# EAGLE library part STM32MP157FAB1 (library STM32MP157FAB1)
32-bit Microcontrollers - MCU 16/32-BITS MICROS Source: Datasheet
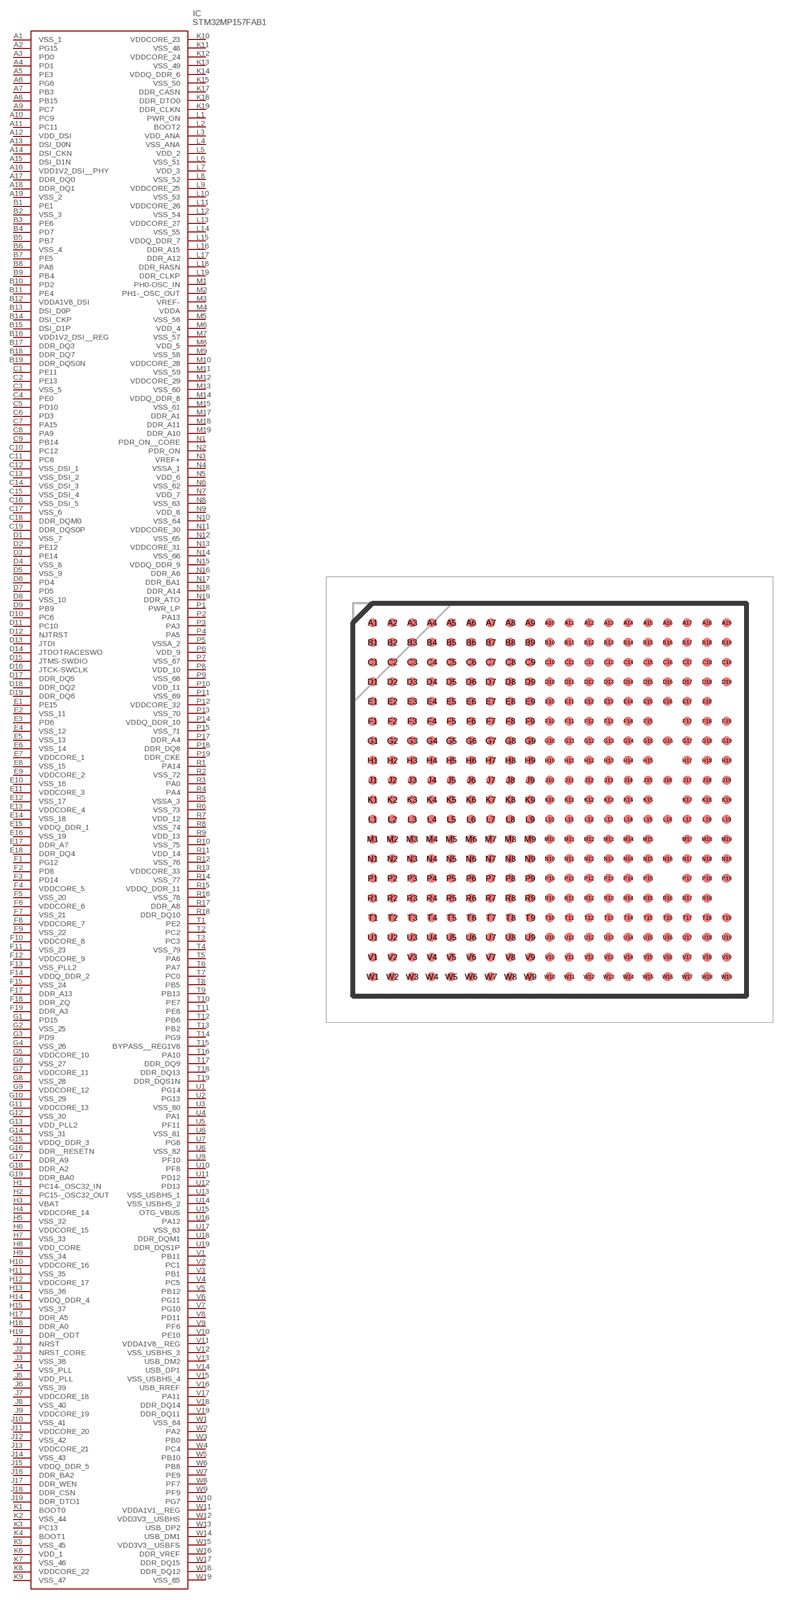
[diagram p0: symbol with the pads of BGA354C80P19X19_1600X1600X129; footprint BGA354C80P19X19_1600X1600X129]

Designator prefix IC

## STM32MP157FAB1 (Description: 32-bit Microcontrollers - MCU 16/32-BITS MICROS; Height: 1.29mm; Manufacturer_Name: STMicroelectronics; Manufacturer_Part_Number: STM32MP157FAB1; Mouser_Part_Number: 511-STM32MP157FAB1; Mouser_Price-Stock: https://www.mouser.co.uk/ProductDetail/STMicroelectronics/STM32MP157FAB1?qs=xZ%2FP%252Ba9zWqaMNhk4KMq8KA%3D%3D)  [BGA354C80P19X19_1600X1600X129]
A1  VSS_1
A2  PG15
A3  PD0
A4  PD1
A5  PE3
A6  PG6
A7  PB3
A8  PB15
A9  PC7
A10  PC9
A11  PC11
A12  VDD_DSI
A13  DSI_D0N
A14  DSI_CKN
A15  DSI_D1N
A16  VDD1V2_DSI__PHY
A17  DDR_DQ0
A18  DDR_DQ1
A19  VSS_2
B1  PE1
B2  VSS_3
B3  PE6
B4  PD7
B5  PB7
B6  VSS_4
B7  PE5
B8  PA8
B9  PB4
B10  PD2
B11  PE4
B12  VDDA1V8_DSI
B13  DSI_D0P
B14  DSI_CKP
B15  DSI_D1P
B16  VDD1V2_DSI__REG
B17  DDR_DQ3
B18  DDR_DQ7
B19  DDR_DQS0N
C1  PE11
C2  PE13
C3  VSS_5
C4  PE0
C5  PD10
C6  PD3
C7  PA15
C8  PA9
C9  PB14
C10  PC12
C11  PC8
C12  VSS_DSI_1
C13  VSS_DSI_2
C14  VSS_DSI_3
C15  VSS_DSI_4
C16  VSS_DSI_5
C17  VSS_6
C18  DDR_DQM0
C19  DDR_DQS0P
D1  VSS_7
D2  PE12
D3  PE14
D4  VSS_8
D5  VSS_9
D6  PD4
D7  PD5
D8  VSS_10
D9  PB9
D10  PC6
D11  PC10
D12  NJTRST
D13  JTDI
D14  JTDOTRACESWO
D15  JTMS-SWDIO
D16  JTCK-SWCLK
D17  DDR_DQ5
D18  DDR_DQ2
D19  DDR_DQ6
E1  PE15
E2  VSS_11
E3  PD6
E4  VSS_12
E5  VSS_13
E6  VSS_14
E7  VDDCORE_1
E8  VSS_15
E9  VDDCORE_2
E10  VSS_16
E11  VDDCORE_3
E12  VSS_17
E13  VDDCORE_4
E14  VSS_18
E15  VDDQ_DDR_1
E16  VSS_19
E17  DDR_A7
E18  DDR_DQ4
F1  PG12
F2  PD8
F3  PD14
F4  VDDCORE_5
F5  VSS_20
F6  VDDCORE_6
F7  VSS_21
F8  VDDCORE_7
F9  VSS_22
F10  VDDCORE_8
F11  VSS_23
F12  VDDCORE_9
F13  VSS_PLL2
F14  VDDQ_DDR_2
F15  VSS_24
F17  DDR_A13
F18  DDR_ZQ
F19  DDR_A3
G1  PD15
G2  VSS_25
G3  PD9
G4  VSS_26
G5  VDDCORE_10
G6  VSS_27
G7  VDDCORE_11
G8  VSS_28
G9  VDDCORE_12
G10  VSS_29
G11  VDDCORE_13
G12  VSS_30
G13  VDD_PLL2
G14  VSS_31
G15  VDDQ_DDR_3
G16  DDR__RESETN
G17  DDR_A9
G18  DDR_A2
G19  DDR_BA0
H1  PC14-_OSC32_IN
H2  PC15-_OSC32_OUT
H3  VBAT
H4  VDDCORE_14
H5  VSS_32
H6  VDDCORE_15
H7  VSS_33
H8  VDD_CORE
H9  VSS_34
H10  VDDCORE_16
H11  VSS_35
H12  VDDCORE_17
H13  VSS_36
H14  VDDQ_DDR_4
H15  VSS_37
H17  DDR_A5
H18  DDR_A0
H19  DDR__ODT
J1  NRST
J2  NRST_CORE
J3  VSS_38
J4  VSS_PLL
J5  VDD_PLL
J6  VSS_39
J7  VDDCORE_18
J8  VSS_40
J9  VDDCORE_19
J10  VSS_41
J11  VDDCORE_20
J12  VSS_42
J13  VDDCORE_21
J14  VSS_43
J15  VDDQ_DDR_5
J16  DDR_BA2
J17  DDR_WEN
J18  DDR_CSN
J19  DDR_DTO1
K1  BOOT0
K2  VSS_44
K3  PC13
K4  BOOT1
K5  VSS_45
K6  VDD_1
K7  VSS_46
K8  VDDCORE_22
K9  VSS_47
K10  VDDCORE_23
K11  VSS_48
K12  VDDCORE_24
K13  VSS_49
K14  VDDQ_DDR_6
K15  VSS_50
K17  DDR_CASN
K18  DDR_DTO0
K19  DDR_CLKN
L1  PWR_ON
L2  BOOT2
L3  VDD_ANA
L4  VSS_ANA
L5  VDD_2
L6  VSS_51
L7  VDD_3
L8  VSS_52
L9  VDDCORE_25
L10  VSS_53
L11  VDDCORE_26
L12  VSS_54
L13  VDDCORE_27
L14  VSS_55
L15  VDDQ_DDR_7
L16  DDR_A15
L17  DDR_A12
L18  DDR_RASN
L19  DDR_CLKP
M1  PH0-OSC_IN
M2  PH1-_OSC_OUT
M3  VREF-
M4  VDDA
M5  VSS_56
M6  VDD_4
M7  VSS_57
M8  VDD_5
M9  VSS_58
M10  VDDCORE_28
M11  VSS_59
M12  VDDCORE_29
M13  VSS_60
M14  VDDQ_DDR_8
M15  VSS_61
M17  DDR_A1
M18  DDR_A11
M19  DDR_A10
N1  PDR_ON__CORE
N2  PDR_ON
N3  VREF+
N4  VSSA_1
N5  VDD_6
N6  VSS_62
N7  VDD_7
N8  VSS_63
N9  VDD_8
N10  VSS_64
N11  VDDCORE_30
N12  VSS_65
N13  VDDCORE_31
N14  VSS_66
N15  VDDQ_DDR_9
N16  DDR_A6
N17  DDR_BA1
N18  DDR_A14
N19  DDR_ATO
P1  PWR_LP
P2  PA13
P3  PA3
P4  PA5
P5  VSSA_2
P6  VDD_9
P7  VSS_67
P8  VDD_10
P9  VSS_68
P10  VDD_11
P11  VSS_69
P12  VDDCORE_32
P13  VSS_70
P14  VDDQ_DDR_10
P15  VSS_71
P17  DDR_A4
P18  DDR_DQ8
P19  DDR_CKE
R1  PA14
R2  VSS_72
R3  PA0
R4  PA4
R5  VSSA_3
R6  VSS_73
R7  VDD_12
R8  VSS_74
R9  VDD_13
R10  VSS_75
R11  VDD_14
R12  VSS_76
R13  VDDCORE_33
R14  VSS_77
R15  VDDQ_DDR_11
R16  VSS_78
R17  DDR_A8
R18  DDR_DQ10
T1  PE2
T2  PC2
T3  PC3
T4  VSS_79
T5  PA6
T6  PA7
T7  PC0
T8  PB5
T9  PB13
T10  PE7
T11  PE8
T12  PB6
T13  PB2
T14  PG9
T15  BYPASS__REG1V8
T16  PA10
T17  DDR_DQ9
T18  DDR_DQ13
T19  DDR_DQS1N
U1  PG14
U2  PG13
U3  VSS_80
U4  PA1
U5  PF11
U6  VSS_81
U7  PG8
U8  VSS_82
U9  PF10
U10  PF8
U11  PD12
U12  PD13
U13  VSS_USBHS_1
U14  VSS_USBHS_2
U15  OTG_VBUS
U16  PA12
U17  VSS_83
U18  DDR_DQM1
U19  DDR_DQS1P
V1  PB11
V2  PC1
V3  PB1
V4  PC5
V5  PB12
V6  PG11
V7  PG10
V8  PD11
V9  PF6
V10  PE10
V11  VDDA1V8__REG
V12  VSS_USBHS_3
V13  USB_DM2
V14  USB_DP1
V15  VSS_USBHS_4
V16  USB_RREF
V17  PA11
V18  DDR_DQ14
V19  DDR_DQ11
W1  VSS_84
W2  PA2
W3  PB0
W4  PC4
W5  PB10
W6  PB8
W7  PE9
W8  PF7
W9  PF9
W10  PG7
W11  VDDA1V1__REG
W12  VDD3V3__USBHS
W13  USB_DP2
W14  USB_DM1
W15  VDD3V3__USBFS
W16  DDR_VREF
W17  DDR_DQ15
W18  DDR_DQ12
W19  VSS_85

## Footprint BGA354C80P19X19_1600X1600X129 (pad centres in mm)
LFBGA - 354balls, 16x16 mm, 0.8 mm pitch, low profile fine pitch ball grid array package outline
smd 0.37 x 0.37: A1 -7.2,7.2; A2 -6.4,7.2; A3 -5.6,7.2; A4 -4.8,7.2; A5 -4,7.2; A6 -3.2,7.2; A7 -2.4,7.2; A8 -1.6,7.2; A9 -0.8,7.2; A10 0,7.2; A11 0.8,7.2; A12 1.6,7.2; A13 2.4,7.2; A14 3.2,7.2; A15 4,7.2; A16 4.8,7.2; A17 5.6,7.2; A18 6.4,7.2; A19 7.2,7.2; B1 -7.2,6.4; B2 -6.4,6.4; B3 -5.6,6.4; B4 -4.8,6.4; B5 -4,6.4; B6 -3.2,6.4; B7 -2.4,6.4; B8 -1.6,6.4; B9 -0.8,6.4; B10 0,6.4; B11 0.8,6.4; B12 1.6,6.4; B13 2.4,6.4; B14 3.2,6.4; B15 4,6.4; B16 4.8,6.4; B17 5.6,6.4; B18 6.4,6.4; B19 7.2,6.4; C1 -7.2,5.6; C2 -6.4,5.6; C3 -5.6,5.6; C4 -4.8,5.6; C5 -4,5.6; C6 -3.2,5.6; C7 -2.4,5.6; C8 -1.6,5.6; C9 -0.8,5.6; C10 0,5.6; C11 0.8,5.6; C12 1.6,5.6; C13 2.4,5.6; C14 3.2,5.6; C15 4,5.6; C16 4.8,5.6; C17 5.6,5.6; C18 6.4,5.6; C19 7.2,5.6; D1 -7.2,4.8; D2 -6.4,4.8; D3 -5.6,4.8; D4 -4.8,4.8; D5 -4,4.8; D6 -3.2,4.8; D7 -2.4,4.8; D8 -1.6,4.8; D9 -0.8,4.8; D10 0,4.8; D11 0.8,4.8; D12 1.6,4.8; D13 2.4,4.8; D14 3.2,4.8; D15 4,4.8; D16 4.8,4.8; D17 5.6,4.8; D18 6.4,4.8; D19 7.2,4.8; E1 -7.2,4; E2 -6.4,4; E3 -5.6,4; E4 -4.8,4; E5 -4,4; E6 -3.2,4; E7 -2.4,4; E8 -1.6,4; E9 -0.8,4; E10 0,4; E11 0.8,4; E12 1.6,4; E13 2.4,4; E14 3.2,4; E15 4,4; E16 4.8,4; E17 5.6,4; E18 6.4,4; F1 -7.2,3.2; F2 -6.4,3.2; F3 -5.6,3.2; F4 -4.8,3.2; F5 -4,3.2; F6 -3.2,3.2; F7 -2.4,3.2; F8 -1.6,3.2; F9 -0.8,3.2; F10 0,3.2; F11 0.8,3.2; F12 1.6,3.2; F13 2.4,3.2; F14 3.2,3.2; F15 4,3.2; F17 5.6,3.2; F18 6.4,3.2; F19 7.2,3.2; G1 -7.2,2.4; G2 -6.4,2.4; G3 -5.6,2.4; G4 -4.8,2.4; G5 -4,2.4; G6 -3.2,2.4; G7 -2.4,2.4; G8 -1.6,2.4; G9 -0.8,2.4; G10 0,2.4; G11 0.8,2.4; G12 1.6,2.4; G13 2.4,2.4; G14 3.2,2.4; G15 4,2.4; G16 4.8,2.4; G17 5.6,2.4; G18 6.4,2.4; G19 7.2,2.4; H1 -7.2,1.6; H2 -6.4,1.6; H3 -5.6,1.6; H4 -4.8,1.6; H5 -4,1.6; H6 -3.2,1.6; H7 -2.4,1.6; H8 -1.6,1.6; H9 -0.8,1.6; H10 0,1.6; H11 0.8,1.6; H12 1.6,1.6; H13 2.4,1.6; H14 3.2,1.6; H15 4,1.6; H17 5.6,1.6; H18 6.4,1.6; H19 7.2,1.6; J1 -7.2,0.8; J2 -6.4,0.8; J3 -5.6,0.8; J4 -4.8,0.8; J5 -4,0.8; J6 -3.2,0.8; J7 -2.4,0.8; J8 -1.6,0.8; J9 -0.8,0.8; J10 0,0.8; J11 0.8,0.8; J12 1.6,0.8; J13 2.4,0.8; J14 3.2,0.8; J15 4,0.8; J16 4.8,0.8; J17 5.6,0.8; J18 6.4,0.8; J19 7.2,0.8; K1 -7.2,0; K2 -6.4,0; K3 -5.6,0; K4 -4.8,0; K5 -4,0; K6 -3.2,0; K7 -2.4,0; K8 -1.6,0; K9 -0.8,0; K10 0,0; K11 0.8,0; K12 1.6,0; K13 2.4,0; K14 3.2,0; K15 4,0; K17 5.6,0; K18 6.4,0; K19 7.2,0; L1 -7.2,-0.8; L2 -6.4,-0.8; L3 -5.6,-0.8; L4 -4.8,-0.8; L5 -4,-0.8; L6 -3.2,-0.8; L7 -2.4,-0.8; L8 -1.6,-0.8; L9 -0.8,-0.8; L10 0,-0.8; L11 0.8,-0.8; L12 1.6,-0.8; L13 2.4,-0.8; L14 3.2,-0.8; L15 4,-0.8; L16 4.8,-0.8; L17 5.6,-0.8; L18 6.4,-0.8; L19 7.2,-0.8; M1 -7.2,-1.6; M2 -6.4,-1.6; M3 -5.6,-1.6; M4 -4.8,-1.6; M5 -4,-1.6; M6 -3.2,-1.6; M7 -2.4,-1.6; M8 -1.6,-1.6; M9 -0.8,-1.6; M10 0,-1.6; M11 0.8,-1.6; M12 1.6,-1.6; M13 2.4,-1.6; M14 3.2,-1.6; M15 4,-1.6; M17 5.6,-1.6; M18 6.4,-1.6; M19 7.2,-1.6; N1 -7.2,-2.4; N2 -6.4,-2.4; N3 -5.6,-2.4; N4 -4.8,-2.4; N5 -4,-2.4; N6 -3.2,-2.4; N7 -2.4,-2.4; N8 -1.6,-2.4; N9 -0.8,-2.4; N10 0,-2.4; N11 0.8,-2.4; N12 1.6,-2.4; N13 2.4,-2.4; N14 3.2,-2.4; N15 4,-2.4; N16 4.8,-2.4; N17 5.6,-2.4; N18 6.4,-2.4; N19 7.2,-2.4; P1 -7.2,-3.2; P2 -6.4,-3.2; P3 -5.6,-3.2; P4 -4.8,-3.2; P5 -4,-3.2; P6 -3.2,-3.2; P7 -2.4,-3.2; P8 -1.6,-3.2; P9 -0.8,-3.2; P10 0,-3.2; P11 0.8,-3.2; P12 1.6,-3.2; P13 2.4,-3.2; P14 3.2,-3.2; P15 4,-3.2; P17 5.6,-3.2; P18 6.4,-3.2; P19 7.2,-3.2; R1 -7.2,-4; R2 -6.4,-4; R3 -5.6,-4; R4 -4.8,-4; R5 -4,-4; R6 -3.2,-4; R7 -2.4,-4; R8 -1.6,-4; R9 -0.8,-4; R10 0,-4; R11 0.8,-4; R12 1.6,-4; R13 2.4,-4; R14 3.2,-4; R15 4,-4; R16 4.8,-4; R17 5.6,-4; R18 6.4,-4; T1 -7.2,-4.8; T2 -6.4,-4.8; T3 -5.6,-4.8; T4 -4.8,-4.8; T5 -4,-4.8; T6 -3.2,-4.8; T7 -2.4,-4.8; T8 -1.6,-4.8; T9 -0.8,-4.8; T10 0,-4.8; T11 0.8,-4.8; T12 1.6,-4.8; T13 2.4,-4.8; T14 3.2,-4.8; T15 4,-4.8; T16 4.8,-4.8; T17 5.6,-4.8; T18 6.4,-4.8; T19 7.2,-4.8; U1 -7.2,-5.6; U2 -6.4,-5.6; U3 -5.6,-5.6; U4 -4.8,-5.6; U5 -4,-5.6; U6 -3.2,-5.6; U7 -2.4,-5.6; U8 -1.6,-5.6; U9 -0.8,-5.6; U10 0,-5.6; U11 0.8,-5.6; U12 1.6,-5.6; U13 2.4,-5.6; U14 3.2,-5.6; U15 4,-5.6; U16 4.8,-5.6; U17 5.6,-5.6; U18 6.4,-5.6; U19 7.2,-5.6; V1 -7.2,-6.4; V2 -6.4,-6.4; V3 -5.6,-6.4; V4 -4.8,-6.4; V5 -4,-6.4; V6 -3.2,-6.4; V7 -2.4,-6.4; V8 -1.6,-6.4; V9 -0.8,-6.4; V10 0,-6.4; V11 0.8,-6.4; V12 1.6,-6.4; V13 2.4,-6.4; V14 3.2,-6.4; V15 4,-6.4; V16 4.8,-6.4; V17 5.6,-6.4; V18 6.4,-6.4; V19 7.2,-6.4; W1 -7.2,-7.2; W2 -6.4,-7.2; W3 -5.6,-7.2; W4 -4.8,-7.2; W5 -4,-7.2; W6 -3.2,-7.2; W7 -2.4,-7.2; W8 -1.6,-7.2; W9 -0.8,-7.2; W10 0,-7.2; W11 0.8,-7.2; W12 1.6,-7.2; W13 2.4,-7.2; W14 3.2,-7.2; W15 4,-7.2; W16 4.8,-7.2; W17 5.6,-7.2; W18 6.4,-7.2; W19 7.2,-7.2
